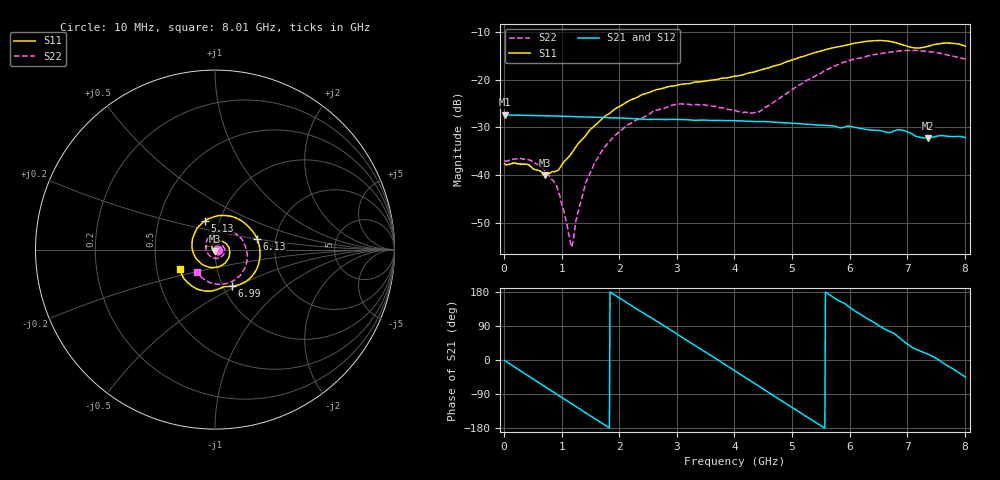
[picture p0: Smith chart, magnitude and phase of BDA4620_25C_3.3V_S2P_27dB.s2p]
!Agilent Technologies,E5071B,MY42404982,A.09.10
!Date: Wed May 06 08:54:41 2026
!Data & Calibration Information:
!Freq	S11:SOLT2(ON)	S21:SOLT2(ON)	S12:SOLT2(ON)	S22:SOLT2(ON)
# Hz S RI R 50
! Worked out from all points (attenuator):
!   801 points, 10 MHz to 8.01 GHz, reference 50 ohm
!   highest |S21| = -27.38 dB at 20 MHz (marker M1); lowest = -32.3 dB at 7.36 GHz (marker M2)
!   lowest |S11| = -40.1 dB at 710 MHz (marker M3), VSWR 1.02, Z = 49.9 - j0.985 ohm
!   |S11| at or under -10 dB: start of sweep to end of sweep
!   |S22| runs from -54.9 to -13.9 dB; largest |S21 - S12| = 0.00021
!   S11 on the Smith chart (normalised r, x): 10 MHz: 1.03, -0.00; 5.13 GHz: 0.85, +0.28; 6.13 GHz: 1.60, +0.20; 6.99 GHz: 1.10, -0.47; 8.01 GHz: 0.66, -0.15
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1e7  0.0132 -0.000809  0.0428 -0.000904  0.0428 -0.000903  0.014 -0.000462
2e7  0.0129 -0.000822  0.0428 -0.00153  0.0428 -0.00171  0.0141 -0.000321
4.4e8  0.0086 -0.00928  0.0304 -0.0291  0.0305 -0.0292  0.0135 -0.0051
7.1e8  -0.00102 -0.00987  0.0141 -0.0394  0.0141 -0.0395  0.00867 -0.00716
9.3e8  -0.00966 -0.00556  -0.00135 -0.0414  -0.00141 -0.0415  0.00356 -0.00626
1.16e9  -0.0157 0.00513  -0.017 -0.0374  -0.017 -0.0375  -0.00142 -0.00123
1.2e9  -0.0164 0.00741  -0.0195 -0.0361  -0.0195 -0.0362  -0.00205 -4.63e-06
1.35e9  -0.0167 0.0166  -0.0277 -0.0299  -0.0278 -0.0299  -0.00358 0.00451
1.53e9  -0.0124 0.0286  -0.0351 -0.02  -0.0352 -0.02  -0.0034 0.0112
1.77e9  0.000908 0.0419  -0.0398 -0.00447  -0.0398 -0.0045  0.000686 0.0204
2.14e9  0.0346 0.0471  -0.0343 0.0194  -0.0343 0.0194  0.0164 0.0291
2.68e9  0.0788 0.00764  -0.00625 0.0378  -0.00627 0.0379  0.0442 0.0196
3.08e9  0.0753 -0.048  0.0185 0.0334  0.0187 0.0333  0.0552 -0.00707
4.01e9  -0.0688 -0.0838  0.0325 -0.0179  0.0325 -0.0179  -0.0101 -0.0465
4.43e9  -0.1247 -0.00638  0.0128 -0.034  0.0128 -0.0341  -0.0446 -0.0117
5.13e9  -0.0553 0.1612  -0.0256 -0.0232  -0.0257 -0.0233  -0.014 0.0865
5.35e9  0.00978 0.1873  -0.0315 -0.0121  -0.0315 -0.0121  0.0227 0.1017
6.13e9  0.2353 0.0584  -0.0182 0.0254  -0.0182 0.0254  0.162 0.036
6.68e9  0.1939 -0.1607  0.00655 0.0271  0.00659 0.0272  0.1701 -0.0901
6.99e9  0.0929 -0.2037  0.0206 0.0197  0.0208 0.0197  0.1263 -0.1566
7.36e9  0.011 -0.2219  0.0235 0.00641  0.0236 0.00648  0.0381 -0.1929
8.01e9  -0.1937 -0.1106  0.0175 -0.0174  0.0176 -0.0174  -0.1015 -0.1275
